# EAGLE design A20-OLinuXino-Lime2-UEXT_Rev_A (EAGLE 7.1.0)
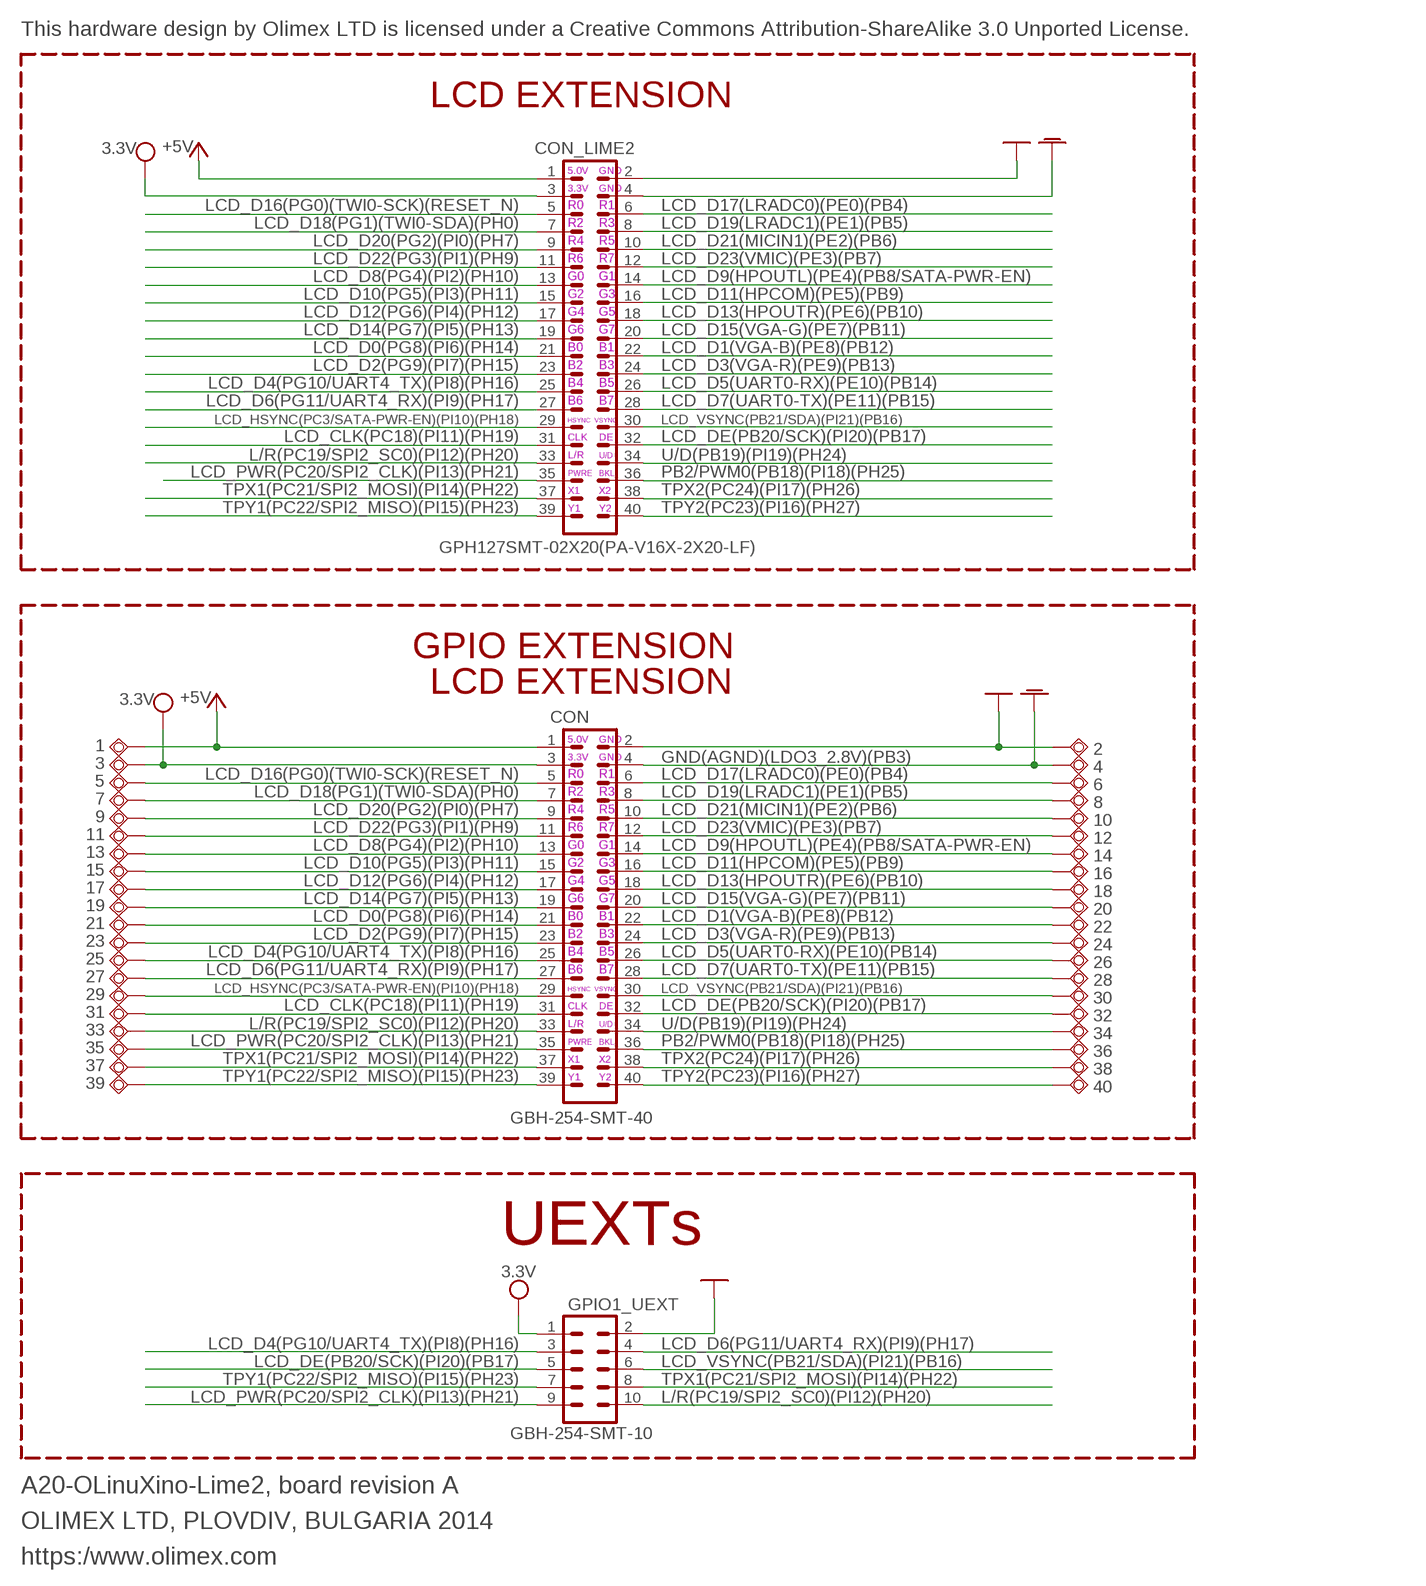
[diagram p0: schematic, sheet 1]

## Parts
1  TESTPAD3  [TEST_PAD40/70/SQUARE]
2  TESTPAD40/70  [TESTPAD]
3  TESTPAD40/70  [TESTPAD]
4  TESTPAD40/70  [TESTPAD]
5  TESTPAD40/70  [TESTPAD]
6  TESTPAD40/70  [TESTPAD]
7  TESTPAD40/70  [TESTPAD]
8  TESTPAD40/70  [TESTPAD]
9  TESTPAD40/70  [TESTPAD]
10  TESTPAD40/70  [TESTPAD]
11  TESTPAD40/70  [TESTPAD]
12  TESTPAD40/70  [TESTPAD]
13  TESTPAD40/70  [TESTPAD]
14  TESTPAD40/70  [TESTPAD]
15  TESTPAD40/70  [TESTPAD]
16  TESTPAD40/70  [TESTPAD]
17  TESTPAD40/70  [TESTPAD]
18  TESTPAD40/70  [TESTPAD]
19  TESTPAD40/70  [TESTPAD]
20  TESTPAD40/70  [TESTPAD]
21  TESTPAD40/70  [TESTPAD]
22  TESTPAD40/70  [TESTPAD]
23  TESTPAD40/70  [TESTPAD]
24  TESTPAD40/70  [TESTPAD]
25  TESTPAD40/70  [TESTPAD]
26  TESTPAD40/70  [TESTPAD]
27  TESTPAD40/70  [TESTPAD]
28  TESTPAD40/70  [TESTPAD]
29  TESTPAD40/70  [TESTPAD]
30  TESTPAD40/70  [TESTPAD]
31  TESTPAD40/70  [TESTPAD]
32  TESTPAD40/70  [TESTPAD]
33  TESTPAD40/70  [TESTPAD]
34  TESTPAD40/70  [TESTPAD]
35  TESTPAD40/70  [TESTPAD]
36  TESTPAD40/70  [TESTPAD]
37  TESTPAD40/70  [TESTPAD]
38  TESTPAD40/70  [TESTPAD]
39  TESTPAD40/70  [TESTPAD]
40  TESTPAD40/70  [TESTPAD]
CON  GBH-254-SMT-40  ML40-GBH-254-SMT-40  [ML40-MALE(GBH-254-SMT-40)]
CON_LIME2  GPH127SMT-02X20(PA-V16X-2X20-LF)  ML40-GPH127SMT-02X20(PA-V16X-2X20-LF)  [GPH127SMT-02X20(PA-V16X-2X20-LF)]
GPIO1_UEXT  GBH-254-SMT-10  ML10MD  [ML10_S]

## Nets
+5V: 1.P$1(PP) CON.1 CON_LIME2.1
GND [PWR]: 2.P$1(PP) CON.2 CON_LIME2.2 GPIO1_UEXT.2
GNDA: 4.P$1(PP) CON.4 CON_LIME2.4
L/R(PC19/SPI2_SC0)(PI12)(PH20): 33.P$1(PP) CON.33 CON_LIME2.33 GPIO1_UEXT.10
LCD_CLK(PC18)(PI11)(PH19): 31.P$1(PP) CON.31 CON_LIME2.31
LCD_D0(PG8)(PI6)(PH14): 21.P$1(PP) CON.21 CON_LIME2.21
LCD_D1(VGA-B)(PE8)(PB12): 22.P$1(PP) CON.22 CON_LIME2.22
LCD_D2(PG9)(PI7)(PH15): 23.P$1(PP) CON.23 CON_LIME2.23
LCD_D3(VGA-R)(PE9)(PB13): 24.P$1(PP) CON.24 CON_LIME2.24
LCD_D4(PG10/UART4_TX)(PI8)(PH16): 25.P$1(PP) CON.25 CON_LIME2.25 GPIO1_UEXT.3
LCD_D5(UART0-RX)(PE10)(PB14): 26.P$1(PP) CON.26 CON_LIME2.26
LCD_D6(PG11/UART4_RX)(PI9)(PH17): 27.P$1(PP) CON.27 CON_LIME2.27 GPIO1_UEXT.4
LCD_D7(UART0-TX)(PE11)(PB15): 28.P$1(PP) CON.28 CON_LIME2.28
LCD_D8(PG4)(PI2)(PH10): 13.P$1(PP) CON.13 CON_LIME2.13
LCD_D9(HPOUTL)(PE4)(PB8/SATA-PWR-EN): 14.P$1(PP) CON.14 CON_LIME2.14
LCD_D10(PG5)(PI3)(PH11): 15.P$1(PP) CON.15 CON_LIME2.15
LCD_D11(HPCOM)(PE5)(PB9): 16.P$1(PP) CON.16 CON_LIME2.16
LCD_D12(PG6)(PI4)(PH12): 17.P$1(PP) CON.17 CON_LIME2.17
LCD_D13(HPOUTR)(PE6)(PB10): 18.P$1(PP) CON.18 CON_LIME2.18
LCD_D14(PG7)(PI5)(PH13): 19.P$1(PP) CON.19 CON_LIME2.19
LCD_D15(VGA-G)(PE7)(PB11): 20.P$1(PP) CON.20 CON_LIME2.20
LCD_D16(PG0)(TWI0-SCK)(RESET_N): 5.P$1(PP) CON.5 CON_LIME2.5
LCD_D17(LRADC0)(PE0)(PB4): 6.P$1(PP) CON.6 CON_LIME2.6
LCD_D18(PG1)(TWI0-SDA)(PH0): 7.P$1(PP) CON.7 CON_LIME2.7
LCD_D19(LRADC1)(PE1)(PB5): 8.P$1(PP) CON.8 CON_LIME2.8
LCD_D20(PG2)(PI0)(PH7): 9.P$1(PP) CON.9 CON_LIME2.9
LCD_D21(MICIN1)(PE2)(PB6): 10.P$1(PP) CON.10 CON_LIME2.10
LCD_D22(PG3)(PI1)(PH9): 11.P$1(PP) CON.11 CON_LIME2.11
LCD_D23(VMIC)(PE3)(PB7): 12.P$1(PP) CON.12 CON_LIME2.12
LCD_DE(PB20/SCK)(PI20)(PB17): 32.P$1(PP) CON.32 CON_LIME2.32 GPIO1_UEXT.5
LCD_HSYNC(PC3/SATA-PWR-EN)(PI10)(PH18): 29.P$1(PP) CON.29 CON_LIME2.29
LCD_PWR(PC20/SPI2_CLK)(PI13)(PH21): 35.P$1(PP) CON.35 CON_LIME2.35 GPIO1_UEXT.9
LCD_VSYNC(PB21/SDA)(PI21)(PB16): 30.P$1(PP) CON.30 CON_LIME2.30 GPIO1_UEXT.6
PB2/PWM0(PB18)(PI18)(PH25): 36.P$1(PP) CON.36 CON_LIME2.36
TPX1(PC21/SPI2_MOSI)(PI14)(PH22): 37.P$1(PP) CON.37 CON_LIME2.37 GPIO1_UEXT.8
TPX2(PC24)(PI17)(PH26): 38.P$1(PP) CON.38 CON_LIME2.38
TPY1(PC22/SPI2_MISO)(PI15)(PH23): 39.P$1(PP) CON.39 CON_LIME2.39 GPIO1_UEXT.7
TPY2(PC23)(PI16)(PH27): 40.P$1(PP) CON.40 CON_LIME2.40
U/D(PB19)(PI19)(PH24): 34.P$1(PP) CON.34 CON_LIME2.34
VCC [PWR]: 3.P$1(PP) CON.3 CON_LIME2.3 GPIO1_UEXT.1 ; supply symbol labelled 3.3V

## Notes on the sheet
- This hardware design by Olimex LTD is licensed under a Creative Commons Attribution-ShareAlike 3.0 Unported License.
- LCD EXTENSION
- 5.0V | GND
- 3.3V | GND
- R0 | R1
- R2 | R3
- R4 | R5
- R6 | R7
- G0 | G1
- G2 | G3
- G4 | G5
- G6 | G7
- B0 | B1
- B2 | B3
- B4 | B5
- B6 | B7
- HSYNC | VSYNC
- CLK | DE
- L/R | U/D
- PWRE | BKL
- X1 | X2
- Y1 | Y2
- GPIO EXTENSION
- LCD EXTENSION
- 5.0V | GND
- 3.3V | GND | GND(AGND)(LDO3_2.8V)(PB3)
- R0 | R1
- R2 | R3
- R4 | R5
- R6 | R7
- G0 | G1
- G2 | G3
- G4 | G5
- G6 | G7
- B0 | B1
- B2 | B3
- B4 | B5
- B6 | B7
- HSYNC | VSYNC
- CLK | DE
- L/R | U/D
- PWRE | BKL
- X1 | X2
- Y1 | Y2
- UEXTs
- A20-OLinuXino-Lime2, board revision A
- OLIMEX LTD, PLOVDIV, BULGARIA 2014
- https:/www.olimex.com

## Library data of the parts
1-40 = gogo:TESTPAD: drill 40mils, diameter 70mils
CON CON_LIME2 = con-harting-ml:ML40: HARTING
GPIO1_UEXT = con-harting-ml:ML10: HARTING

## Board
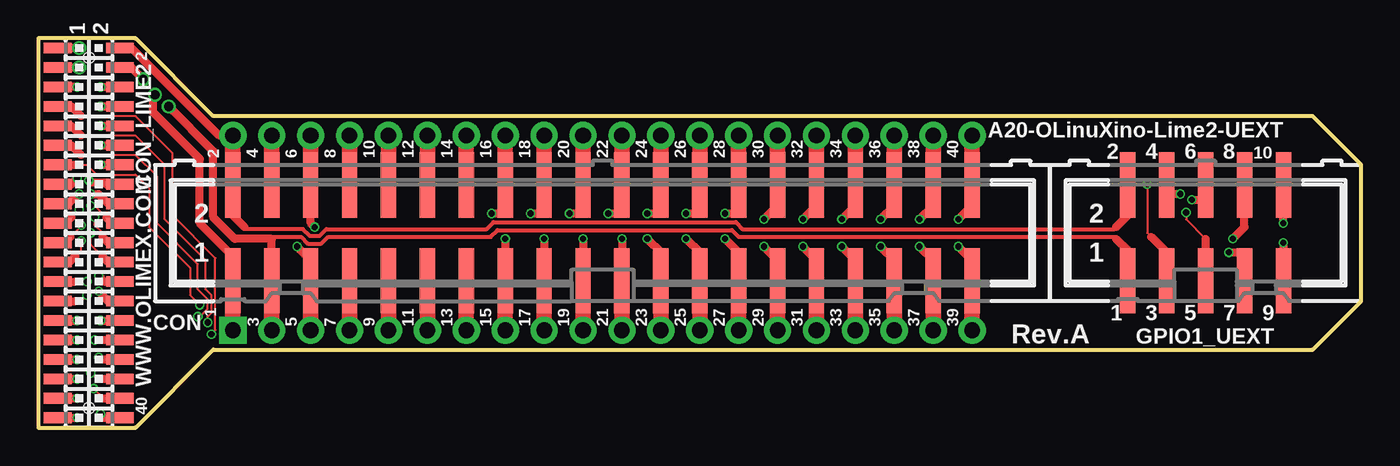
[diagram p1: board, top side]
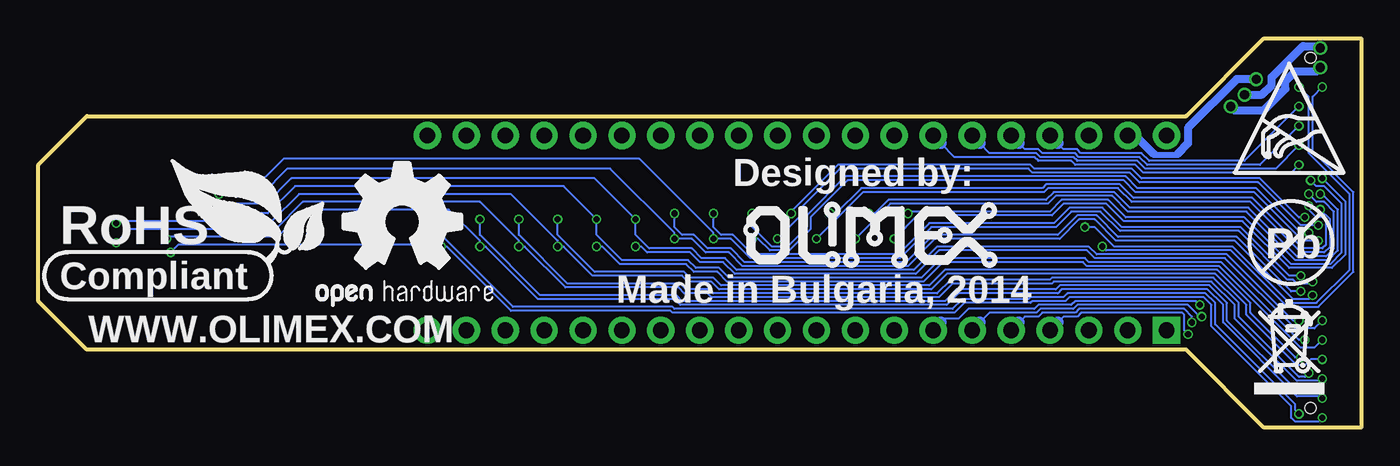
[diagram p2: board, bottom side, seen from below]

Size 86.36 x 25.4 mm. Coordinates in mm from the lower left corner, seen from the top.
Outline: 0,0 6.35,0 11.43,5.08 83.19,5.08 86.36,8.26 86.36,17.14 83.19,20.32 11.43,20.32 6.35,25.4 0,25.4 0,0
Copper layers (1*16): Top 0.035mm / dielectric 1.5mm / Bottom 0.035mm
Design rules "default": minimum track width 4.5mil, minimum drill 10mil, track to track 5mil, track to pad 5mil, pad to pad 5mil, via to via 5mil, smd to smd 1mil, copper to edge 10mil, drill to drill 8mil, minimum pad ring 6mil, minimum via ring 4mil, stop-mask expansion 4mil, vias tented up to drill 25mil, thermal gap 12mil

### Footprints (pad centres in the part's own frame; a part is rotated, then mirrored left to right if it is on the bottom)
TEST_PAD40/70/SQUARE = drill 1.016 pad 1.778 square: P$1 0,0
TESTPAD = drill 1.016 pad 1.778: P$1 0,0
ML40-MALE(GBH-254-SMT-40) = smd 1 x 4.25: 1 -24.13,-3.125; 2 -24.13,3.125; 3 -21.59,-3.125; 4 -21.59,3.125; 5 -19.05,-3.125; 6 -19.05,3.125; 7 -16.51,-3.125; 8 -16.51,3.125; 9 -13.97,-3.125; 10 -13.97,3.125; 11 -11.43,-3.125; 12 -11.43,3.125; 13 -8.89,-3.125; 14 -8.89,3.125; 15 -6.35,-3.125; 16 -6.35,3.125; 17 -3.81,-3.125; 18 -3.81,3.125; 19 -1.27,-3.125; 20 -1.27,3.125; 21 1.27,-3.125; 22 1.27,3.125; 23 3.81,-3.125; 24 3.81,3.125; 25 6.35,-3.125; 26 6.35,3.125; 27 8.89,-3.125; 28 8.89,3.125; 29 11.43,-3.125; 30 11.43,3.125; 31 13.97,-3.125; 32 13.97,3.125; 33 16.51,-3.125; 34 16.51,3.125; 35 19.05,-3.125; 36 19.05,3.125; 37 21.59,-3.125; 38 21.59,3.125; 39 24.13,-3.125; 40 24.13,3.125
GPH127SMT-02X20(PA-V16X-2X20-LF) = smd 0.7 x 1.8: 1 -12.065,-2.032; 2 -12.065,2.032; 3 -10.795,-2.032; 4 -10.795,2.032; 5 -9.525,-2.032; 6 -9.525,2.032; 7 -8.255,-2.032; 8 -8.255,2.032; 9 -6.985,-2.032; 10 -6.985,2.032; 11 -5.715,-2.032; 12 -5.715,2.032; 13 -4.445,-2.032; 14 -4.445,2.032; 15 -3.175,-2.032; 16 -3.175,2.032; 17 -1.905,-2.032; 18 -1.905,2.032; 19 -0.635,-2.032; 20 -0.635,2.032; 21 0.635,-2.032; 22 0.635,2.032; 23 1.905,-2.032; 24 1.905,2.032; 25 3.175,-2.032; 26 3.175,2.032; 27 4.445,-2.032; 28 4.445,2.032; 29 5.715,-2.032; 30 5.715,2.032; 31 6.985,-2.032; 32 6.985,2.032; 33 8.255,-2.032; 34 8.255,2.032; 35 9.525,-2.032; 36 9.525,2.032; 37 10.795,-2.032; 38 10.795,2.032; 39 12.065,-2.032; 40 12.065,2.032 | hole 0.7: -11.43,0; 11.43,0
ML10_S = smd 1 x 4.25: 1 -5.08,-3.125; 2 -5.08,3.125; 3 -2.54,-3.125; 4 -2.54,3.125; 5 0,-3.125; 6 0,3.125; 7 2.54,-3.125; 8 2.54,3.125; 9 5.08,-3.125; 10 5.08,3.125

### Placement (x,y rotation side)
1  12.7,6.35 0 top
2  12.7,19.05 90 top
3  15.24,6.35 90 top
4  15.24,19.05 90 top
5  17.78,6.35 90 top
6  17.78,19.05 90 top
7  20.32,6.35 90 top
8  20.32,19.05 90 top
9  22.86,6.35 90 top
10  22.86,19.05 90 top
11  25.4,6.35 90 top
12  25.4,19.05 90 top
13  27.94,6.35 90 top
14  27.94,19.05 90 top
15  30.48,6.35 90 top
16  30.48,19.05 90 top
17  33.02,6.35 90 top
18  33.02,19.05 90 top
19  35.56,6.35 90 top
20  35.56,19.05 90 top
21  38.1,6.35 90 top
22  38.1,19.05 90 top
23  40.64,6.35 90 top
24  40.64,19.05 90 top
25  43.18,6.35 90 top
26  43.18,19.05 90 top
27  45.72,6.35 90 top
28  45.72,19.05 90 top
29  48.26,6.35 90 top
30  48.26,19.05 90 top
31  50.8,6.35 90 top
32  50.8,19.05 90 top
33  53.34,6.35 90 top
34  53.34,19.05 90 top
35  55.88,6.35 90 top
36  55.88,19.05 90 top
37  58.42,6.35 90 top
38  58.42,19.05 90 top
39  60.96,6.35 90 top
40  60.96,19.05 90 top
CON  36.83,12.7 0 top
CON_LIME2  3.3,12.7 270 top
GPIO1_UEXT  76.2,12.7 0 top
U$5  [LOGO-OPENHARDWARE_8X8]  62.61,13.34 0 bottom
U$6  [OLIMEX1_V]  22.61,10.29 0 bottom
U$9  [PB]  4.57,12.06 0 bottom
U$10  [ESD_SYMBOL]  8.26,16.64 0 bottom
U$11  [RECYCLE_BIN1/8]  6.99,2.16 0 bottom
U$12  [ROHS]  84.96,9.02 0 bottom

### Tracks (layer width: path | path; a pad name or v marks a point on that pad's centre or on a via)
+5V  (via drill 0.6)
  Top 0.508: CON.1 12.7,11.18 10.54,13.34 10.54,17.53 7.49,20.57 7.49,21.59 v7.62,21.72 | v2.67,24.77 CON_LIME2.1
  Top 1.016: 1.P$1 CON.1
  Bottom 0.508: v2.67,24.77 2.79,24.89 3.81,24.89 5.84,22.86 5.84,22.35 6.48,21.72 v7.62,21.72
GND
  Top 0.254: 13.46,13.08 13.59,12.95 17.27,12.95 17.72,12.51 18.35,12.51 18.8,12.95 29.27,12.95 29.72,13.4 45.53,13.4 45.97,12.95 70.23,12.95 70.36,13.08
  Top 0.508: CON.2 12.7,13.84 13.46,13.08 | GPIO1_UEXT.2 71.12,13.84 70.36,13.08 | CON_LIME2.2 6.1,24.77 11.81,19.05 2.P$1
  Top 1.016: CON.2 2.P$1
GNDA  (via drill 0.6)
  Top 0.508: CON_LIME2.4 6.1,23.5 v6.86,22.73
  Top 1.016: 4.P$1 CON.4
  Bottom 0.381: 12,17.84 12.06,17.78 13.46,17.78 13.53,17.84
  Bottom 0.508: 12,17.84 11.3,18.54 11.3,19.56 8.13,22.73 v6.86,22.73 | 13.53,17.84 14.73,19.05 4.P$1
L/R(PC19/SPI2_SC0)(PI12)(PH20)  (via drill 0.4)
  Top 0.508: v52.45,11.81 53.34,10.92 CON.33 | v81.28,13.34 GPIO1_UEXT.10 | CON_LIME2.33 v2.54,4.45
  Top 1.016: CON.33 33.P$1
  Bottom 0.127: v2.54,4.45 3.3,4.45 3.68,4.06 4.19,4.06 7.49,7.37 7.49,8 9.53,10.03 27.05,10.03 28.07,9.02 41.91,9.02 42.42,9.53 43.94,9.53 44.32,9.91 50.16,9.91 52.07,11.81 v52.45,11.81 52.45,12.19 55.5,15.24 69.34,15.24 71.12,13.46 81.15,13.46 v81.28,13.34
LCD_CLK(PC18)(PI11)(PH19)  (via drill 0.4)
  Top 0.508: CON_LIME2.31 v2.54,5.71 | v49.91,11.81 50.8,10.92 CON.31
  Top 1.016: CON.31 31.P$1
  Bottom 0.127: v2.54,5.71 3.05,5.21 3.94,5.21 9.27,10.54 17.91,10.54 18.16,10.79 27.3,10.79 28.57,9.53 41.4,9.53 42.04,10.16 43.56,10.16 44.07,10.67 48.39,10.67 49.53,11.81 v49.91,11.81
LCD_D0(PG8)(PI6)(PH14)  (via drill 0.4)
  Top 0.127: 2.1,12.45 2.79,13.14 v2.79,13.21 | CON.21 38.1,9.53
  Top 0.508: CON_LIME2.21 1.71,12.06 2.1,12.45 | v38.1,12.32 CON.21
  Top 1.016: CON.21 21.P$1
  Bottom 0.127: v2.79,13.21 3.94,13.21 6.73,16 14.48,16 15.11,16.64 21.46,16.64 21.72,16.89 34.04,16.89 36.7,14.22 36.7,13.72 v38.1,12.32
LCD_D1(VGA-B)(PE8)(PB12)  (via drill 0.4)
  Top 0.127: v3.68,13.72 3.68,13.21 4.19,12.7 4.19,12.45
  Top 0.508: 4.19,12.45 4.57,12.06 CON_LIME2.22 | v37.21,13.97 38.1,13.97 CON.22
  Top 1.016: CON.22 22.P$1
  Bottom 0.127: v3.68,13.72 4.06,13.72 6.6,16.26 14.35,16.26 14.99,16.89 21.34,16.89 21.59,17.14 34.16,17.14 37.21,14.1 v37.21,13.97
LCD_D2(PG9)(PI7)(PH15)  (via drill 0.4)
  Top 0.127: 2.41,11.18 2.79,11.56 v2.79,12.19
  Top 0.508: CON_LIME2.23 2.03,10.79 2.41,11.18 | v39.75,12.32 40.64,11.43 40.64,9.53
  Top 1.016: 23.P$1 40.64,9.53 CON.23
  Bottom 0.127: v2.79,12.19 3.81,12.19 6.99,15.37 14.73,15.37 15.49,16.13 33.53,16.13 35.94,13.72 35.94,12.95 37.34,11.56 38.61,11.56 39.37,12.32 v39.75,12.32
LCD_D3(VGA-R)(PE9)(PB13)  (via drill 0.4)
  Top 0.127: 4.19,11.18 3.43,11.94 v3.43,12.7
  Top 0.508: 4.19,11.18 4.57,10.79 CON_LIME2.24 | v39.75,13.97 40.64,13.97 CON.24
  Top 1.016: CON.24 24.P$1
  Bottom 0.127: v3.43,12.7 3.94,12.7 6.86,15.62 14.61,15.62 15.37,16.38 33.66,16.38 36.2,13.84 36.2,13.08 37.47,11.81 38.48,11.81 39.75,13.08 v39.75,13.97
LCD_D4(PG10/UART4_TX)(PI8)(PH16)  (via drill 0.4)
  Top 0.127: v72.39,15.88 72.39,12.7 72.64,12.45 | 2.41,9.53 v3.17,9.53
  Top 0.508: 73.66,9.53 GPIO1_UEXT.3 73.66,11.43 72.64,12.45 | CON_LIME2.25 2.41,9.53 | v42.29,12.32 43.18,11.43 CON.25
  Top 1.016: CON.25 25.P$1
  Bottom 0.127: v3.17,9.53 3.3,9.4 4.19,9.4 4.45,9.65 4.83,9.65 8,12.83 15.75,12.83 17.02,14.1 18.92,14.1 19.94,13.08 28.07,13.08 30.1,11.05 39.88,11.05 41.15,12.32 v42.29,12.32 42.29,12.7 47.12,17.53 70.36,17.53 72.01,15.88 v72.39,15.88
LCD_D5(UART0-RX)(PE10)(PB14)  (via drill 0.4)
  Top 0.508: v3.94,9.91 4.32,9.53 CON_LIME2.26 | v42.29,13.97 43.18,13.97 CON.26
  Top 1.016: CON.26 26.P$1
  Bottom 0.127: v3.94,9.91 4.7,9.91 7.87,13.08 15.62,13.08 16.89,14.35 19.05,14.35 20.07,13.34 28.19,13.34 30.23,11.3 39.75,11.3 41.02,12.57 41.78,12.57 42.29,13.08 v42.29,13.97
LCD_D6(PG11/UART4_RX)(PI9)(PH17)  (via drill 0.4)
  Top 0.127: 2.41,8.26 2.79,8.26 v3.17,8.64
  Top 0.508: GPIO1_UEXT.4 73.66,15.24 v74.55,15.24 | CON_LIME2.27 2.41,8.26 | v44.83,12.32 45.72,11.43 CON.27
  Top 1.016: CON.27 27.P$1
  Bottom 0.127: v3.17,8.64 3.43,8.38 4.45,8.38 8.26,12.19 16,12.19 17.4,13.59 18.41,13.59 19.68,12.32 27.81,12.32 29.59,10.54 40.39,10.54 41.27,11.43 42.8,11.43 43.69,12.32 v44.83,12.32 44.83,12.7 49.02,16.89 70.1,16.89 71.75,15.24 v74.55,15.24
LCD_D7(UART0-TX)(PE11)(PB15)  (via drill 0.4)
  Top 0.127: 4.83,8.26 CON_LIME2.28
  Top 0.508: v3.94,8.89 4.57,8.26 4.83,8.26 | v44.83,13.97 45.72,13.97 CON.28
  Top 1.016: CON.28 28.P$1
  Bottom 0.127: v3.94,8.89 4.57,8.89 8.13,12.45 15.88,12.45 17.27,13.84 18.54,13.84 19.81,12.57 27.94,12.57 29.72,10.79 40.26,10.79 41.15,11.68 42.67,11.68 43.56,12.57 44.32,12.57 44.83,13.08 v44.83,13.97
LCD_D8(PG4)(PI2)(PH10)  (via drill 0.4)
  Top 0.127: v10.54,8 9.91,8.64 9.91,10.41 7.24,13.08 7.24,15.62 6.35,16.51 3.81,16.51 3.17,17.14 2.41,17.14
  Top 0.508: CON_LIME2.13 2.41,17.14
  Top 1.016: 13.P$1 CON.13
  Bottom 0.127: v10.54,8 10.79,8.26 18.67,8.26 18.92,8 21.08,8 21.34,7.75 25.65,7.75 26.29,7.11 27.18,7.11 27.43,6.86
  Bottom 0.762: 27.43,6.86 13.P$1
LCD_D9(HPOUTL)(PE4)(PB8/SATA-PWR-EN)  (via drill 0.4)
  Top 0.508: v4.06,17.14 CON_LIME2.14
  Top 1.016: 14.P$1 CON.14
  Bottom 0.127: v4.06,17.14 4.57,16.64 14.22,16.64 14.73,17.14 18.67,17.14 18.92,17.4 21.08,17.4 21.34,17.65 26.54,17.65 27.43,18.54
  Bottom 0.762: 27.43,18.54 14.P$1
LCD_D10(PG5)(PI3)(PH11)  (via drill 0.4)
  Top 0.508: v2.54,16.26 2.16,15.88 CON_LIME2.15 | v30.48,12.32 CON.15
  Top 1.016: CON.15 15.P$1
  Bottom 0.127: v2.54,16.26 1.02,14.73 1.02,11.3 1.91,10.41 4.7,10.41 7.75,13.46 15.49,13.46 16.64,14.61 19.43,14.61 20.19,13.84 28.96,13.84 v30.48,12.32
LCD_D11(HPCOM)(PE5)(PB9)  (via drill 0.4)
  Top 0.508: v3.3,16.13 3.43,16 4.32,16 4.45,15.88 CON_LIME2.16 | CON.16 30.48,13.97 v29.59,13.97
  Top 1.016: CON.16 16.P$1
  Bottom 0.127: v3.3,16.13 2.92,15.75 2.41,15.75 1.27,14.61 1.27,11.43 2.03,10.67 4.57,10.67 7.62,13.72 15.37,13.72 16.51,14.86 19.56,14.86 20.32,14.1 29.46,14.1 v29.59,13.97
LCD_D12(PG6)(PI4)(PH12)  (via drill 0.4)
  Top 0.508: v2.67,15.24 2.6,15.24 1.97,14.61 CON_LIME2.17 | v33.02,12.32 CON.17
  Top 1.016: CON.17 17.P$1
  Bottom 0.127: v2.67,15.24 2.54,15.24 1.52,14.22 1.52,11.56 2.16,10.92 4.32,10.92 7.49,14.1 15.24,14.1 16.26,15.11 19.94,15.11 20.45,14.61 30.73,14.61 v33.02,12.32
LCD_D13(HPOUTR)(PE6)(PB10)  (via drill 0.4)
  Top 0.508: v3.43,15.24 3.94,15.24 4.57,14.61 CON_LIME2.18 | v32.13,13.97 33.02,13.97 CON.18
  Top 1.016: CON.18 18.P$1
  Bottom 0.127: v3.43,15.24 2.92,14.73 2.41,14.73 1.78,14.1 1.78,11.68 2.29,11.18 4.19,11.18 7.37,14.35 15.11,14.35 16.13,15.37 20.07,15.37 20.57,14.86 30.86,14.86 31.75,13.97 v32.13,13.97
LCD_D14(PG7)(PI5)(PH13)  (via drill 0.4)
  Top 0.127: v2.67,14.22 2.16,13.72
  Top 0.508: 2.16,13.72 1.78,13.34 CON_LIME2.19 | v35.56,12.32 CON.19
  Top 1.016: CON.19 19.P$1
  Bottom 0.127: v2.67,14.22 2.03,13.59 2.03,11.81 2.41,11.43 3.94,11.43 7.24,14.73 14.99,14.73 15.88,15.62 20.45,15.62 20.7,15.37 32.38,15.37 32.51,15.37 v35.56,12.32
LCD_D15(VGA-G)(PE7)(PB11)  (via drill 0.4)
  Top 0.127: v3.43,14.48 3.68,14.48 4.45,13.72
  Top 0.508: 4.45,13.72 4.83,13.34 CON_LIME2.20 | v34.67,13.97 35.56,13.97 CON.20
  Top 1.016: CON.20 20.P$1
  Bottom 0.127: v3.43,14.48 3.43,14.22 2.92,13.72 2.54,13.72 2.29,13.46 2.29,11.94 2.54,11.68 3.81,11.68 7.11,14.99 14.86,14.99 15.75,15.88 20.57,15.88 20.83,15.62 32.64,15.62 34.29,13.97 v34.67,13.97
LCD_D16(PG0)(TWI0-SCK)(RESET_N)  (via drill 0.4)
  Top 0.508: v2.54,22.23 CON_LIME2.5 | CON.5 17.78,10.92 v16.89,11.81
  Top 1.016: CON.5 5.P$1
  Bottom 0.127: v2.54,22.23 3.17,21.59 3.17,18.03 0.51,15.37 0.51,10.16 2.79,7.87 4.83,7.87 8.51,11.56 16.64,11.56 v16.89,11.81
LCD_D17(LRADC0)(PE0)(PB4)  (via drill 0.4)
  Top 0.508: v4.06,22.23 CON_LIME2.6 | v18.03,13.08 17.78,13.34 CON.6
  Top 1.016: CON.6 6.P$1
  Bottom 0.127: v4.06,22.23 3.43,21.59 3.43,17.91 0.76,15.24 0.76,10.29 2.92,8.13 4.7,8.13 8.38,11.81 16.13,11.81 17.4,13.08 v18.03,13.08
LCD_D18(PG1)(TWI0-SDA)(PH0)  (via drill 0.4)
  Top 0.127: v11.3,6.1 11.56,6.35 11.56,11.05 8.76,13.84 8.76,17.91 6.35,20.32 2.79,20.32
  Top 0.508: CON_LIME2.7 2.16,20.95 2.79,20.32
  Top 1.016: 7.P$1 CON.7
  Bottom 0.127: v11.3,6.1 11.56,6.35 11.56,7.37 11.68,7.49 18.29,7.49 18.54,7.24 19.43,7.24 19.81,6.86
  Bottom 0.762: 19.81,6.86 7.P$1
LCD_D19(LRADC1)(PE1)(PB5)  (via drill 0.4)
  Top 0.508: v4.06,20.95 CON_LIME2.8
  Top 1.016: 8.P$1 CON.8
  Bottom 0.127: v4.06,20.95 7.62,17.4 13.84,17.4 14.35,17.91 18.29,17.91 18.54,18.16 19.43,18.16 19.81,18.54
  Bottom 0.762: 19.81,18.54 8.P$1
LCD_D20(PG2)(PI0)(PH7)  (via drill 0.4)
  Top 0.127: v11.05,6.86 11.05,7.24 11.3,7.49 11.3,8.64 10.92,9.02 10.92,10.92 8.26,13.59 8.26,17.14 6.35,19.05 2.79,19.05
  Top 0.508: CON_LIME2.9 2.16,19.68 2.79,19.05
  Top 1.016: 9.P$1 CON.9
  Bottom 0.127: v11.05,6.86 11.05,7.24 11.56,7.75 18.41,7.75 18.67,7.49 20.83,7.49 21.08,7.24 21.97,7.24 22.35,6.86
  Bottom 0.762: 22.35,6.86 9.P$1
LCD_D21(MICIN1)(PE2)(PB6)  (via drill 0.4)
  Top 0.508: v4.06,19.68 CON_LIME2.10
  Top 1.016: 10.P$1 CON.10
  Bottom 0.127: v4.06,19.68 6.6,17.14 13.97,17.14 14.48,17.65 18.41,17.65 18.67,17.91 20.83,17.91 21.08,18.16 21.97,18.16 22.35,18.54
  Bottom 0.762: 22.35,18.54 10.P$1
LCD_D22(PG3)(PI1)(PH9)  (via drill 0.4)
  Top 0.127: v10.41,7.24 10.54,7.24 11.05,7.75 11.05,8.38 10.41,9.02 10.41,10.67 7.75,13.34 7.75,16.38 6.35,17.78 2.79,17.78
  Top 0.508: CON_LIME2.11 2.16,18.41 2.79,17.78
  Top 1.016: 11.P$1 CON.11
  Bottom 0.127: v10.41,7.24 10.54,7.24 11.3,8 18.54,8 18.8,7.75 20.95,7.75 21.21,7.49 24.26,7.49 24.89,6.86
  Bottom 0.762: 24.89,6.86 11.P$1
LCD_D23(VMIC)(PE3)(PB7)  (via drill 0.4)
  Top 0.508: v4.06,18.41 CON_LIME2.12
  Top 1.016: 12.P$1 CON.12
  Bottom 0.127: v4.06,18.41 5.59,16.89 14.1,16.89 14.61,17.4 18.54,17.4 18.8,17.65 20.95,17.65 21.21,17.91 24.26,17.91 24.89,18.54
  Bottom 0.762: 24.89,18.54 12.P$1
LCD_DE(PB20/SCK)(PI20)(PB17)  (via drill 0.4)
  Top 0.127: v74.93,14.03 74.93,13.59 76.2,12.32
  Top 0.508: v49.91,13.59 50.8,14.48 CON.32 | 76.2,12.32 GPIO1_UEXT.5 | v3.68,5.71 CON_LIME2.32
  Top 1.016: CON.32 32.P$1
  Bottom 0.127: v3.68,5.71 4.06,5.71 9.14,10.79 17.78,10.79 18.03,11.05 27.43,11.05 28.7,9.78 41.27,9.78 41.91,10.41 43.43,10.41 43.94,10.92 48.26,10.92 49.91,12.57 v49.91,13.59 52.07,15.75 69.6,15.75 71.37,13.97 74.87,13.97 v74.93,14.03
LCD_HSYNC(PC3/SATA-PWR-EN)(PI10)(PH18)  (via drill 0.4)
  Top 0.508: CON_LIME2.29 v2.54,6.99 | v47.37,11.81 48.26,10.92 CON.29
  Top 1.016: CON.29 29.P$1
  Bottom 0.127: v2.54,6.99 3.05,6.48 4.32,6.48 8.89,11.05 17.4,11.05 17.91,11.56 27.56,11.56 29.08,10.03 40.89,10.03 41.66,10.79 43.18,10.79 43.81,11.43 46.61,11.43 46.99,11.81 v47.37,11.81
LCD_PWR(PC20/SPI2_CLK)(PI13)(PH21)  (via drill 0.4)
  Top 0.508: v54.99,11.81 55.88,10.92 CON.35 | v81.28,12.06 GPIO1_UEXT.9 | CON_LIME2.35 v2.54,3.17
  Top 1.016: CON.35 35.P$1
  Bottom 0.127: v2.54,3.17 2.67,3.05 4.19,3.05 8.26,7.11 8.26,8 9.78,9.53 20.07,9.53 20.19,9.4 26.67,9.4 27.56,8.51 42.42,8.51 42.67,8.76 44.2,8.76 44.58,9.14 51.94,9.14 54.61,11.81 v54.99,11.81 54.99,12.19 57.53,14.73 69.09,14.73 70.87,12.95 80.39,12.95 v81.28,12.06
LCD_VSYNC(PB21/SDA)(PI21)(PB16)  (via drill 0.4)
  Top 0.508: v47.37,13.59 48.26,14.48 CON.30 | GPIO1_UEXT.6 76.2,14.86 v75.31,14.86 | v4.06,6.99 CON_LIME2.30
  Top 1.016: CON.30 30.P$1
  Bottom 0.127: v4.06,6.99 4.45,6.99 8.76,11.3 17.27,11.3 17.78,11.81 27.69,11.81 29.21,10.29 40.77,10.29 41.53,11.05 43.05,11.05 43.69,11.68 46.48,11.68 47.37,12.57 v47.37,13.59 50.04,16.26 69.85,16.26 71.5,14.61 75.06,14.61 v75.31,14.86
PB2/PWM0(PB18)(PI18)(PH25)  (via drill 0.4)
  Top 0.127: v3.43,3.56 3.81,3.17 4.19,3.17
  Top 0.508: 4.19,3.17 CON_LIME2.36 | v54.99,13.59 55.88,14.48 CON.36
  Top 1.016: CON.36 36.P$1
  Bottom 0.127: v3.43,3.56 3.68,3.3 4.06,3.3 8,7.24 8,8.13 9.65,9.78 20.19,9.78 20.32,9.65 26.8,9.65 27.69,8.76 42.29,8.76 42.55,9.02 44.07,9.02 44.45,9.4 51.82,9.4 54.99,12.57 v54.99,13.59
TPX1(PC21/SPI2_MOSI)(PI14)(PH22)  (via drill 0.4)
  Top 0.508: v57.53,11.81 58.42,10.92 CON.37 | v77.98,12.32 78.74,13.08 GPIO1_UEXT.8 | CON_LIME2.37 v2.54,1.91
  Top 1.016: CON.37 37.P$1
  Bottom 0.127: v2.54,1.91 2.67,2.03 4.19,2.03 9.02,6.86 9.02,8 10.03,9.02 19.56,9.02 19.81,8.76 26.29,8.76 27.05,8 44.45,8 44.83,8.38 53.72,8.38 57.15,11.81 v57.53,11.81 57.53,12.19 59.56,14.22 68.96,14.22 70.74,12.45 77.85,12.45 v77.98,12.32
TPX2(PC24)(PI17)(PH26)  (via drill 0.4)
  Top 0.127: 4.25,1.91 v3.62,2.54
  Top 0.508: 4.25,1.91 CON_LIME2.38 | v57.53,13.59 58.42,14.48 CON.38
  Top 1.016: CON.38 38.P$1
  Bottom 0.127: v3.62,2.54 4.32,2.54 8.76,6.99 8.76,8.13 9.91,9.27 19.68,9.27 19.94,9.02 26.42,9.02 27.18,8.26 44.32,8.26 44.7,8.64 53.59,8.64 57.53,12.57 v57.53,13.59
TPY1(PC22/SPI2_MISO)(PI15)(PH23)  (via drill 0.4)
  Top 0.508: v60.07,11.81 60.96,10.92 CON.39 | GPIO1_UEXT.7 78.74,11.43 v77.72,11.43 | CON_LIME2.39 v2.54,0.64
  Top 1.016: CON.39 39.P$1
  Bottom 0.127: v2.54,0.64 2.79,0.38 4.32,0.38 4.57,0.64 4.57,1.4 9.78,6.6 9.78,8 10.29,8.51 19.05,8.51 19.3,8.26 21.46,8.26 21.59,8.13 25.91,8.13 26.54,7.49 44.96,7.49 45.09,7.62 55.5,7.62 59.69,11.81 v60.07,11.81 60.2,11.94 77.22,11.94 v77.72,11.43
TPY2(PC23)(PI16)(PH27)  (via drill 0.4)
  Top 0.508: CON_LIME2.40 4.32,0.64 v4.06,0.89 | v60.07,13.59 60.96,14.48 CON.40
  Top 1.016: CON.40 40.P$1
  Bottom 0.127: v4.06,0.89 4.32,1.14 4.32,1.52 9.53,6.73 9.53,8.13 10.16,8.76 19.18,8.76 19.43,8.51 21.59,8.51 21.72,8.38 26.04,8.38 26.67,7.75 44.83,7.75 44.96,7.87 55.37,7.87 60.07,12.57 v60.07,13.59
U/D(PB19)(PI19)(PH24)  (via drill 0.4)
  Top 0.508: v3.94,4.57 4.06,4.45 CON_LIME2.34 | v52.45,13.59 53.34,14.48 CON.34
  Top 1.016: CON.34 34.P$1
  Bottom 0.127: v3.94,4.57 4.32,4.57 7.24,7.49 7.24,8.13 9.4,10.29 27.18,10.29 28.19,9.27 41.78,9.27 42.29,9.78 43.81,9.78 44.2,10.16 50.04,10.16 52.45,12.57 v52.45,13.59
VCC  (via drill 0.6)
  Top 0.254: 15.24,12.32 15.37,12.45 17.14,12.45 17.59,12 18.48,12 18.92,12.45 29.53,12.45 29.97,12.89 45.28,12.89 45.72,12.45 70.23,12.45 70.36,12.32
  Top 0.508: CON.3 15.24,12.32 12.83,12.32 11.43,13.72 11.43,18.03 v8.51,20.95 | GPIO1_UEXT.1 71.12,11.56 70.36,12.32 | v2.67,23.5 CON_LIME2.3
  Top 1.016: 3.P$1 CON.3
  Bottom 0.508: v2.67,23.5 2.92,23.24 4.32,23.24 4.95,22.61 4.95,22.1 6.35,20.7 8.26,20.7 v8.51,20.95

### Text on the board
tNames: A20-OLinuXino-Lime2-UEXT | 2 | 4 | 6 | 8 | 10 | 1 | 3 | 5 | 7 | 9 | Rev.A | WWW.OLIMEX.COM
bNames: Designed by: | Made in Bulgaria, 2014 | WWW.OLIMEX.COM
